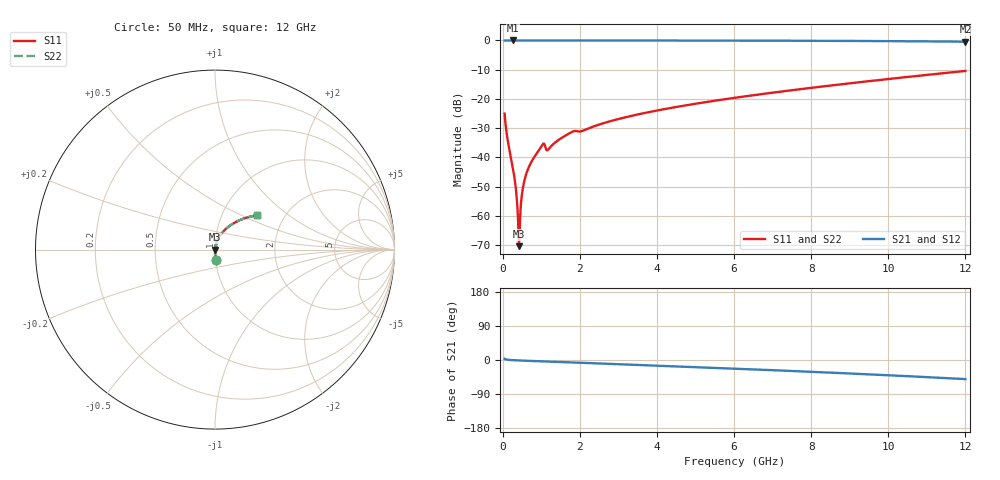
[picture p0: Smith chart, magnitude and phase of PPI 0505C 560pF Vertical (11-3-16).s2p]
# GHz S MA R 50
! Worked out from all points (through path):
!   1601 points, 50 MHz to 12 GHz, reference 50 ohm
!   highest |S21| = 0.00 dB at 266.6 MHz (marker M1); lowest = -0.4 dB at 12 GHz (marker M2)
!   group delay of S21, straight-line fit = 11.6 ps
!   lowest |S11| = -70.4 dB at 423.4 MHz (marker M3), VSWR 1.00, Z = 50 + j0.00266 ohm
!   |S11| at or under -10 dB: start of sweep to end of sweep
!   |S22| runs from -70.4 to -10.4 dB; largest |S21 - S12| = 0
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0.05  0.05589 -86.8  0.9983 3.1  0.9983 3.1  0.05589 -86.8
0.2665938  0.006431 -88.1  0.9997 -0.4  0.9997 -0.4  0.006431 -88.1
0.3263437  0.003534 -86.2  0.9997 -0.7  0.9997 -0.7  0.003534 -86.2
0.3860938  0.001252 -77.6  0.9997 -1.0  0.9997 -1.0  0.001252 -77.6
0.4234375  0.0003019 5.0  0.9997 -1.2  0.9997 -1.2  0.0003019 5.0
0.4607812  0.001222 74.0  0.9997 -1.4  0.9997 -1.4  0.001222 74.0
0.5055937  0.002481 81.0  0.9996 -1.6  0.9996 -1.6  0.002481 81.0
0.528  0.003084 82.3  0.9996 -1.7  0.9996 -1.7  0.003084 82.3
0.6101562  0.005172 84.1  0.9996 -2.0  0.9996 -2.0  0.005172 84.1
0.7445938  0.008352 84.6  0.9995 -2.6  0.9995 -2.6  0.008352 84.6
0.9985312  0.01518 80.5  0.9983 -3.7  0.9983 -3.7  0.01518 80.5
1.058281  0.01717 71.9  0.9956 -3.9  0.9956 -3.9  0.01717 71.9
1.18525  0.01368 76.0  0.9975 -4.1  0.9975 -4.1  0.01368 76.0
1.409312  0.01899 82.3  0.9989 -5.1  0.9989 -5.1  0.01899 82.3
1.752875  0.02629 80.0  0.9979 -6.4  0.9979 -6.4  0.02629 80.0
2.044156  0.02801 77.0  0.9967 -7.4  0.9967 -7.4  0.02801 77.0
2.85825  0.0427 78.4  0.9981 -10.5  0.9981 -10.5  0.0427 78.4
4.038312  0.06393 74.3  0.9969 -15.0  0.9969 -15.0  0.06393 74.3
6.025  0.1045 66.6  0.9932 -22.8  0.9932 -22.8  0.1045 66.6
8.019156  0.155 58.4  0.9863 -31.2  0.9863 -31.2  0.155 58.4
10.01331  0.2193 49.3  0.9737 -40.3  0.9737 -40.3  0.2193 49.3
12  0.3005 39.3  0.9514 -50.4  0.9514 -50.4  0.3005 39.3
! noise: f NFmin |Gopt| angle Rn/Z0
0.05  0.0002914  0.823  0.2023  0.0003454
1.372  0.003593  0.6448  3.77  0.001914
2.701  0.005031  0.5347  7.146  0.001904
4.031  0.006097  0.4575  10.15  0.001873
5.36  0.007437  0.4244  12.99  0.002096
6.682  0.008826  0.4064  15.64  0.002371
8.012  0.0103  0.398  18.15  0.002697
9.341  0.01188  0.3973  20.55  0.003088
10.67  0.01362  0.4035  22.91  0.003569
12  0.01557  0.4159  25.27  0.004172
